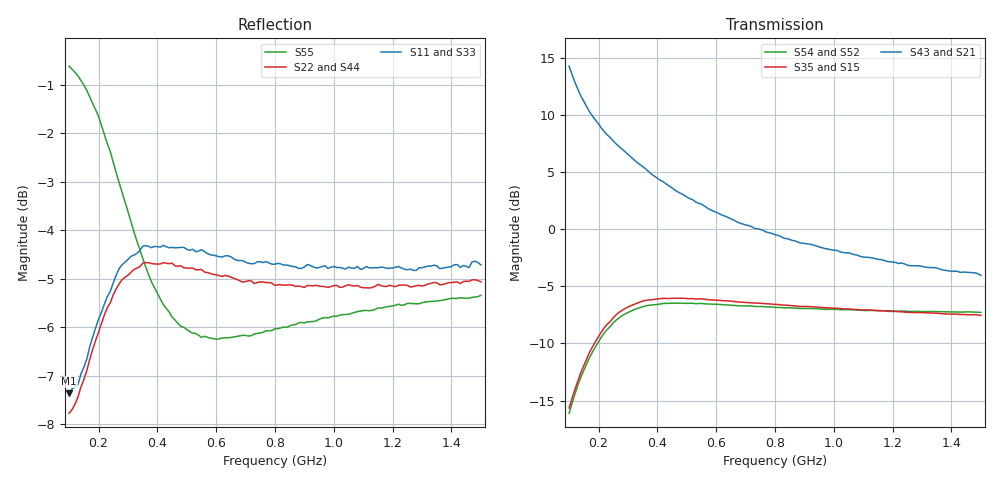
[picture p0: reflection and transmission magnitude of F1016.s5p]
!  POLYFET RF DEVICES
!  S PARAMETERS FOR
!  F1016 (Each Side)
!  VDS=28, IDQ=200mA
! Date: Mon Oct 21 17:40:39 1991
! Bias (V mA) : V1=2.3989000  I1=0.0047421  V2=27.998800  I2=208.57320
!AWR Design Environment (2053) Wed Feb 04 14:40:24 2004
!freq-unit  param-type  data-format  keyword  impedance-ohms
# MHz  S  MA  R  50
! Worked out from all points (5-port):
!   141 points, 100 MHz to 1.5 GHz, reference 50 ohm
!   strongest paths, dB at 100 MHz, 450 MHz, 800 MHz, 1.15 GHz, 1.5 GHz:
!     S43: 14.3, 3.6, -0.5, -2.6, -4.1
!     S21: 14.3, 3.6, -0.5, -2.6, -4.1
!     S35: -15.7, -6.0, -6.6, -7.1, -7.5
!     S15: -15.7, -6.0, -6.6, -7.1, -7.5
!     S54: -16.1, -6.5, -6.8, -7.1, -7.3
!     S52: -16.1, -6.5, -6.8, -7.1, -7.3
!   lowest |S11| = -7.4 dB at 100 MHz (marker M1), VSWR 2.50, Z = 46.2 - j45.4 ohm
!   |S11| at or under -10 dB: nowhere
